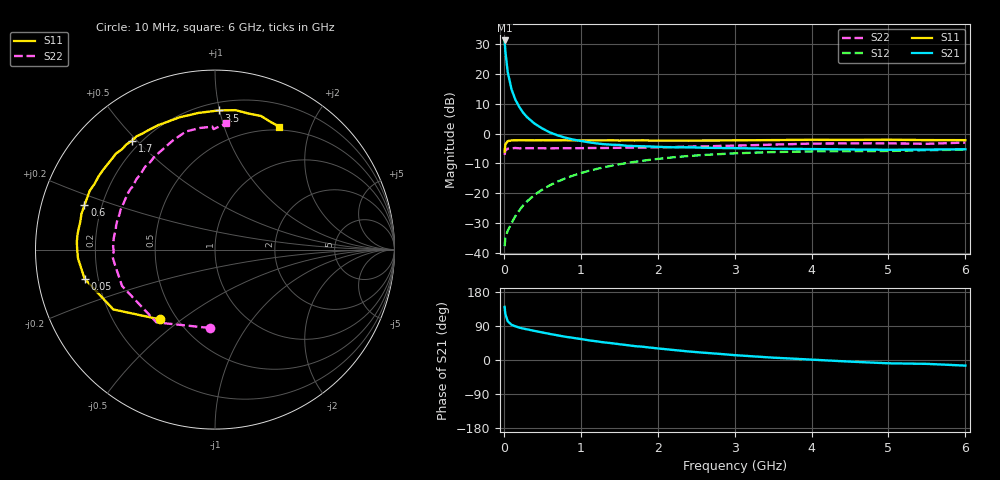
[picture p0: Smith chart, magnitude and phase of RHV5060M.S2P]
! SIEMENS Small Signal Semiconductors
! BFR106
! Si NPN RF Bipolar Junction Transistor in SOT23
! VCE = 0.5 V  IC = 60 mA
! Common Emitter S-Parameters:  August  1996
# GHz  S  MA  R  50
!  f  S11  S21  S12  S22
! GHz  MAG  ANG  MAG  ANG  MAG  ANG  MAG  ANG
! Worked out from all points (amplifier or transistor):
!   36 points, 10 MHz to 6 GHz, reference 50 ohm
!   highest |S21| = 31.2 dB at 10 MHz (marker M1)
!   |S21| within 3 dB of that: start of sweep to 18.26 MHz
!   unconditionally stable (mu >= 1): 68.63 MHz to end of sweep
!   at 250 MHz: K = 1.46, MAG = 11.6 dB, |S12| = -24.2 dB
!   at 1.4 GHz: K = 1.26, MAG = 0.5 dB, |S12| = -10.8 dB
!   at 6 GHz: K = 1.04, MAG = -1.1 dB, |S12| = -5.4 dB
!   S11 on the Smith chart (normalised r, x): 10 MHz: 0.41, -0.42; 50 MHz: 0.15, -0.11; 600 MHz: 0.13, +0.16; 1.7 GHz: 0.17, +0.48; 3.5 GHz: 0.26, +0.99; 6 GHz: 0.46, +1.56
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0.01  0.4946 -128.1  36.33 140.2  0.0129 54.1  0.4376 -93.8
0.02  0.6572 -149.5  23.92 120.8  0.0179 43.0  0.5204 -128.8
0.05  0.7445 -167.4  10.77 102.2  0.0234 42.3  0.556 -158.6
0.1  0.7651 -176.4  5.498 93.1  0.0315 52.2  0.5639 -171.4
0.15  0.7686 179.2  3.69 88.9  0.0412 59.1  0.572 -175.8
0.2  0.7709 176.6  2.801 85.6  0.0511 62.9  0.5643 -179.0
0.25  0.7706 174.3  2.242 83.0  0.062 65.0  0.5678 178.5
0.3  0.7696 172.4  1.891 81.0  0.0724 66.2  0.5681 176.9
0.4  0.7664 168.2  1.463 76.7  0.0939 67.1  0.5679 173.8
0.5  0.7704 165.1  1.213 72.7  0.1146 66.8  0.5662 171.0
0.6  0.7684 161.2  1.041 68.7  0.1357 65.8  0.5639 168.6
0.8  0.7713 154.9  0.85 61.4  0.1769 62.7  0.568 163.8
1.1  0.7656 144.6  0.714 52.0  0.2355 57.1  0.5711 157.3
1.3  0.7649 138.6  0.662 46.6  0.2713 52.8  0.5714 152.6
1.7  0.7632 127.3  0.616 36.6  0.3347 44.7  0.5795 144.3
2.2  0.7621 114.5  0.587 26.5  0.3987 34.6  0.5919 134.1
2.8  0.7631 100.7  0.572 16.2  0.451 23.6  0.6189 122.8
3.5  0.7755 88.5  0.556 6.2  0.4885 12.6  0.6511 111.3
4.5  0.7808 75.9  0.54 -4.3  0.5055 -0.1  0.6828 97.2
5  0.7873 71.0  0.534 -8.7  0.5093 -5.0  0.685 91.2
5.5  0.7754 66.2  0.538 -10.2  0.5243 -7.4  0.6713 90.7
6  0.7734 62.4  0.543 -14.8  0.5369 -13.2  0.7057 85.0
